(* Logix 5000 AddOnInstructionDefinition export YAI_Assy_151_22_23_EIP_Hz; software revision 17.00 *)

ADD_ON_INSTRUCTION YAI_Assy_151_22_23_EIP_Hz   (* revision 1.0, vendor Yaskawa America, Inc. *)
// YAI Assembly 151 and 22/23
// Help:
// This add-on instruction is for use with input assembly 151 and output assemblies 20 or 21.
// Node_Input_Assy is defined as the node's input assembly integer array.
// Node_Output_Assy is defined as the node's output assembly integer array.
VAR_IN_OUT
   Node_Input_Assy : AB:ETHERNET_MODULE_INT_8Bytes:I:0; {required}   // Input assembly words
   Node_Output_Assy : AB:ETHERNET_MODULE_INT_6Bytes:O:0; {required}   // Output assembly words
END_VAR
VAR_INPUT
   RunFwd : BOOL; {visible}   // Forward run command
   RunRev : BOOL; {visible}   // Reverse run command
   FaultReset : BOOL; {visible}   // Fault reset command
   Net_Control : BOOL;   // Network control bit to switch between b1-02 setting and network.
   Net_Ref : BOOL;   // Network reference bit to switch between b1-01 setting and network.
   Freq_Ref : REAL; {visible}   // Frequency reference command in Hz (xx.xx resolution)
END_VAR
VAR_OUTPUT
   Faulted : BOOL; {visible}   // Drive faulted status bit
   Alarm : BOOL; {visible}   // Drive warning (alarm) status bit
   Ready : BOOL; {visible}   // Drive ready status bit
   NetRefStatus : BOOL; {visible}   // Drive network reference status bit (1 = reference coming from network)
   NetCtrlStatus : BOOL; {visible}   // Drive network run source status bit (1 = source coming from network)
   At_Speed : BOOL; {visible}   // Drive at commanded speed status bit
   Output_Freq : REAL; {visible}   // Drive output frequency in Hz (xx.xx resolution)
   Running : BOOL; {visible}
   ZSP : BOOL;
   RunningRev : BOOL; {visible}
   Reset : BOOL;
   OPE : BOOL;
   UV : BOOL;
   MFO_1_Status : BOOL;
   MFO_2_Status : BOOL;
   MFO_3_Status : BOOL;
   ZSV : BOOL;
   Torque_Actual : REAL; {visible}
   Output_Current : REAL; {visible}
END_VAR
VAR_INPUT
   Torq_Ref_Limit : REAL;
   Motor_Rated_Torq : REAL;
END_VAR
VAR
   FRef_Convert : DINT;
   FOut_Convert : REAL;
   FOut_Temp : REAL;
   Fault_Reset_Timer : TIMER := (PRE := 250);
   TOut_Temp : REAL;
   TOut_Convert : REAL;
   IOut_Temp : REAL;
   IOut_Convert : REAL;
   Motor_Torq_Temp : REAL;
   TRef_Convert : REAL;
END_VAR

ROUTINE Logic   (* ladder *)
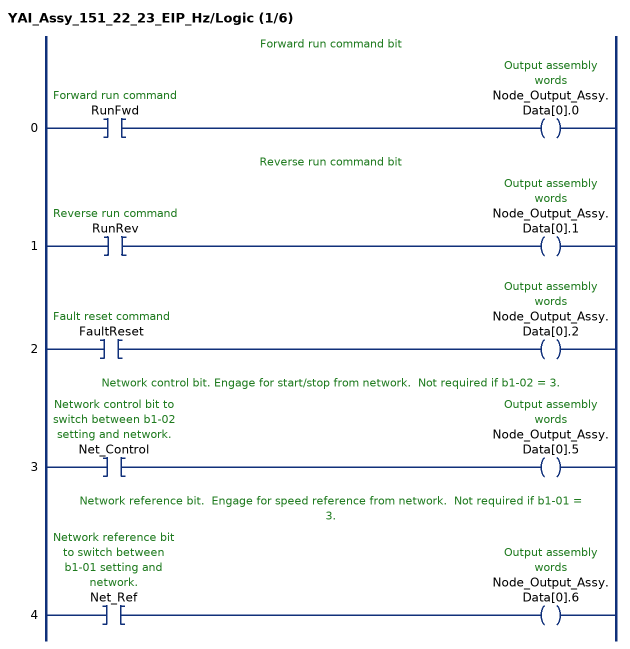
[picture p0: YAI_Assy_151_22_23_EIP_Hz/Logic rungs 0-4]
   // Forward run command bit
   0: XIC(RunFwd)OTE(Node_Output_Assy.Data[0].0);
   // Reverse run command bit
   1: XIC(RunRev)OTE(Node_Output_Assy.Data[0].1);
   2: XIC(FaultReset)OTE(Node_Output_Assy.Data[0].2);
   // Network control bit. Engage for start/stop from network.  Not required if b1-02 = 3.
   3: XIC(Net_Control)OTE(Node_Output_Assy.Data[0].5);
   // Network reference bit.  Engage for speed reference from network.  Not required if b1-01 = 3.
   4: XIC(Net_Ref)OTE(Node_Output_Assy.Data[0].6);
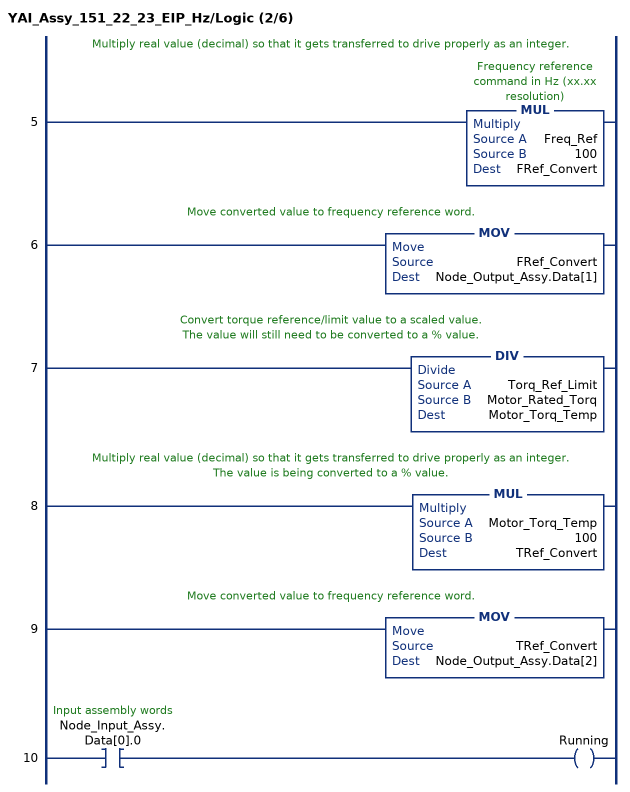
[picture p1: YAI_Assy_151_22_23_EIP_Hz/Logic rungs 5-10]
   // Multiply real value (decimal) so that it gets transferred to drive properly as an integer.
   5: MUL(Freq_Ref,100,FRef_Convert);
   // Move converted value to frequency reference word.
   6: MOV(FRef_Convert,Node_Output_Assy.Data[1]);
   // Convert torque reference/limit value to a scaled value.
   // The value will still need to be converted to a % value.
   7: DIV(Torq_Ref_Limit,Motor_Rated_Torq,Motor_Torq_Temp);
   // Multiply real value (decimal) so that it gets transferred to drive properly as an integer.
   // The value is being converted to a % value.
   8: MUL(Motor_Torq_Temp,100,TRef_Convert);
   // Move converted value to frequency reference word.
   9: MOV(TRef_Convert,Node_Output_Assy.Data[2]);
   10: XIC(Node_Input_Assy.Data[0].0)OTE(Running);
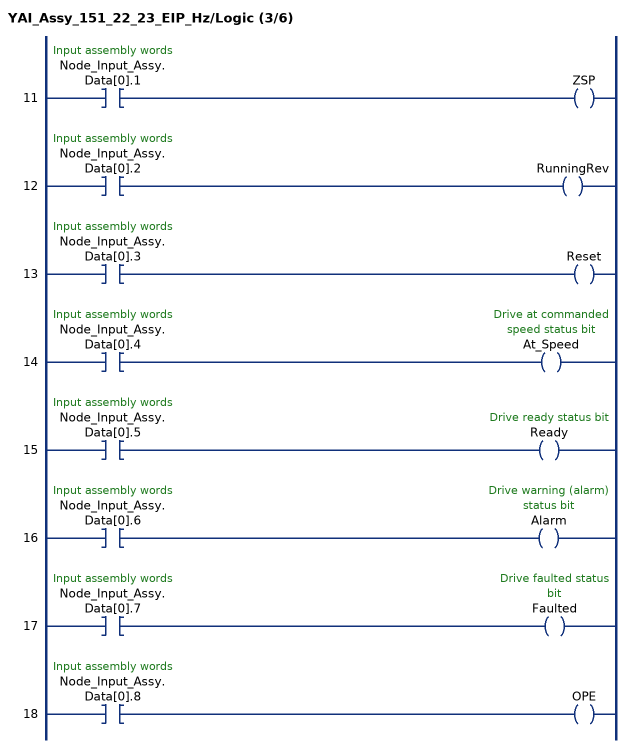
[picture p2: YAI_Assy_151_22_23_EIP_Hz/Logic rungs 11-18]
   11: XIC(Node_Input_Assy.Data[0].1)OTE(ZSP);
   12: XIC(Node_Input_Assy.Data[0].2)OTE(RunningRev);
   13: XIC(Node_Input_Assy.Data[0].3)OTE(Reset);
   14: XIC(Node_Input_Assy.Data[0].4)OTE(At_Speed);
   15: XIC(Node_Input_Assy.Data[0].5)OTE(Ready);
   16: XIC(Node_Input_Assy.Data[0].6)OTE(Alarm);
   17: XIC(Node_Input_Assy.Data[0].7)OTE(Faulted);
   18: XIC(Node_Input_Assy.Data[0].8)OTE(OPE);
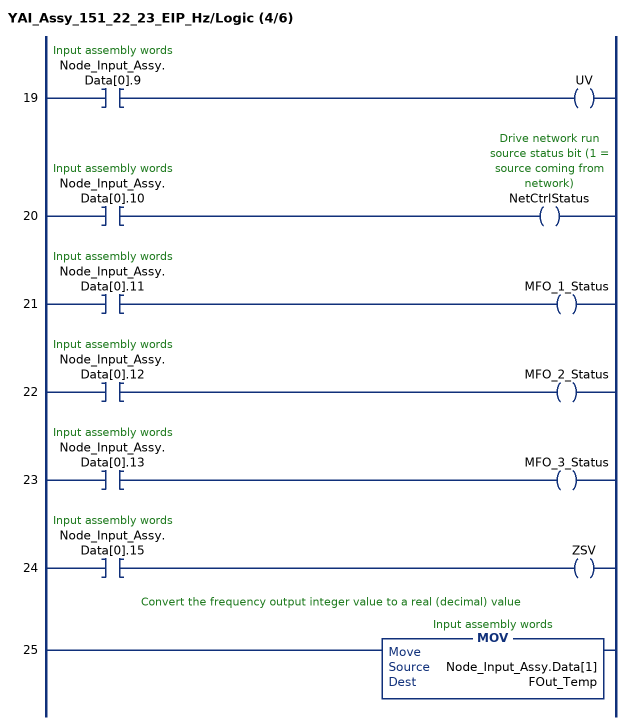
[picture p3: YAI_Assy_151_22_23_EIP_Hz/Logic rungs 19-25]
   19: XIC(Node_Input_Assy.Data[0].9)OTE(UV);
   20: XIC(Node_Input_Assy.Data[0].10)OTE(NetCtrlStatus);
   21: XIC(Node_Input_Assy.Data[0].11)OTE(MFO_1_Status);
   22: XIC(Node_Input_Assy.Data[0].12)OTE(MFO_2_Status);
   23: XIC(Node_Input_Assy.Data[0].13)OTE(MFO_3_Status);
   24: XIC(Node_Input_Assy.Data[0].15)OTE(ZSV);
   // Convert the frequency output integer value to a real (decimal) value
   25: MOV(Node_Input_Assy.Data[1],FOut_Temp);
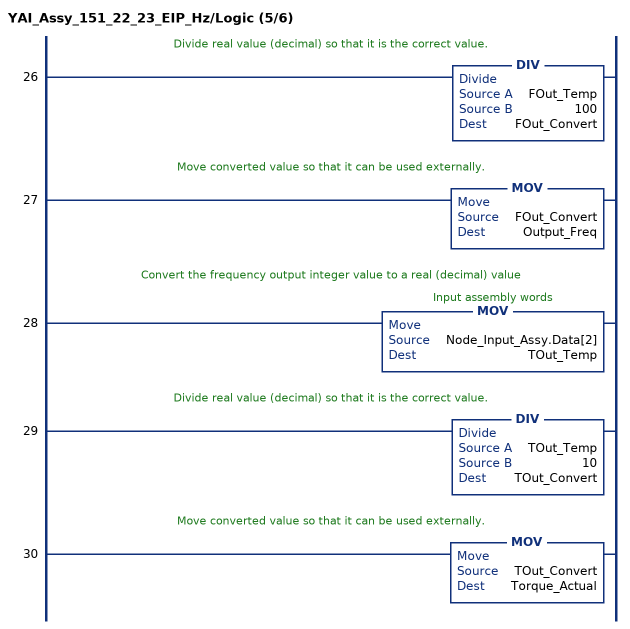
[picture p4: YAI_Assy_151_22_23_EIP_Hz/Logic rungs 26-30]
   // Divide real value (decimal) so that it is the correct value.
   26: DIV(FOut_Temp,100,FOut_Convert);
   // Move converted value so that it can be used externally.
   27: MOV(FOut_Convert,Output_Freq);
   // Convert the frequency output integer value to a real (decimal) value
   28: MOV(Node_Input_Assy.Data[2],TOut_Temp);
   // Divide real value (decimal) so that it is the correct value.
   29: DIV(TOut_Temp,10,TOut_Convert);
   // Move converted value so that it can be used externally.
   30: MOV(TOut_Convert,Torque_Actual);
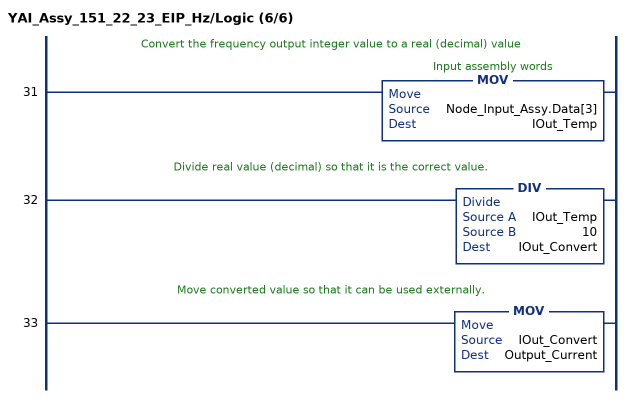
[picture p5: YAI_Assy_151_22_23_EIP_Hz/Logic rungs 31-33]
   // Convert the frequency output integer value to a real (decimal) value
   31: MOV(Node_Input_Assy.Data[3],IOut_Temp);
   // Divide real value (decimal) so that it is the correct value.
   32: DIV(IOut_Temp,10,IOut_Convert);
   // Move converted value so that it can be used externally.
   33: MOV(IOut_Convert,Output_Current);
END_ROUTINE
END_ADD_ON_INSTRUCTION
